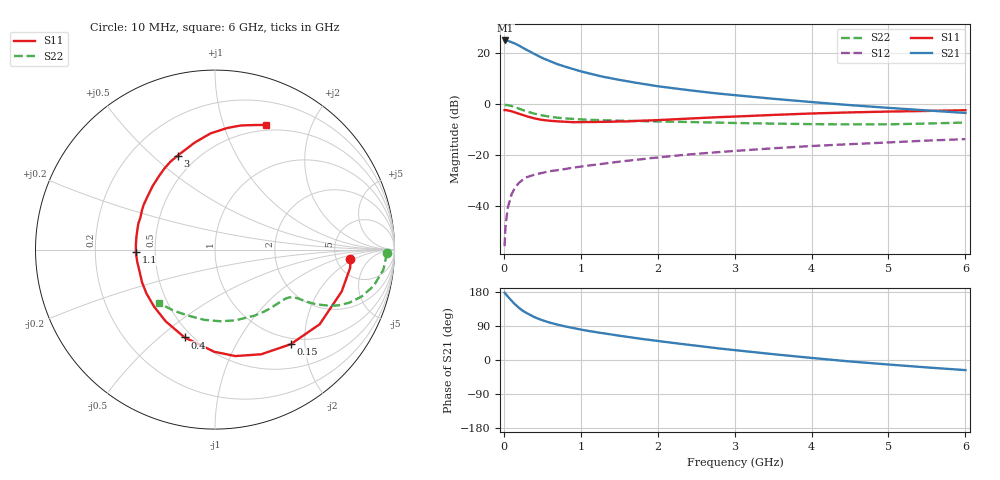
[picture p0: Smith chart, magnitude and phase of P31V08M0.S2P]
! SIEMENS Small Signal Semiconductors
! BFP181
! Si NPN RF Bipolar Junction Transistor in SOT143
! VCE = 1 V  IC = 8 mA
! Common Emitter S-Parameters:  March  1996
# GHz  S  MA  R  50
!  f  S11  S21  S12  S22
! GHz  MAG  ANG  MAG  ANG  MAG  ANG  MAG  ANG
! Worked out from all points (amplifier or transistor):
!   36 points, 10 MHz to 6 GHz, reference 50 ohm
!   highest |S21| = 24.9 dB at 20 MHz (marker M1)
!   |S21| within 3 dB of that: start of sweep to 253.4 MHz
!   unconditionally stable (mu >= 1): 794.9 MHz to end of sweep
!   at 250 MHz: K = 0.40, MSG = 25.9 dB, |S12| = -29.7 dB
!   at 1.4 GHz: K = 1.31, MAG = 13.2 dB, |S12| = -23.1 dB
!   at 6 GHz: K = 1.21, MAG = 2.4 dB, |S12| = -13.8 dB
!   S11 on the Smith chart (normalised r, x): 10 MHz: 6.80, -1.59; 150 MHz: 0.89, -1.72; 400 MHz: 0.46, -0.61; 1.1 GHz: 0.39, -0.01; 3 GHz: 0.39, +0.60; 6 GHz: 0.44, +1.40
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0.01  0.7555 -3.8  17.58 177.7  0.0016 80.5  0.9581 -1.2
0.02  0.76 -7.6  17.65 175.4  0.0037 83.9  0.9538 -2.6
0.05  0.7435 -18.3  17.33 167.9  0.0089 82.4  0.9449 -6.8
0.1  0.7163 -35.5  16.32 156.4  0.0167 72.4  0.9078 -12.8
0.15  0.675 -51.4  15.19 146.1  0.0233 64.2  0.8572 -17.8
0.2  0.6374 -66.2  13.94 137.1  0.0284 59.9  0.8045 -21.6
0.25  0.6039 -79.2  12.57 129.4  0.0326 55.1  0.7531 -24.4
0.3  0.5692 -90.4  11.47 123.5  0.0364 51.6  0.7085 -26.2
0.4  0.5181 -109.1  9.526 112.9  0.0407 47.3  0.6412 -28.4
0.5  0.4848 -124.6  7.989 104.9  0.0441 44.4  0.5929 -29.5
0.6  0.4652 -136.7  6.915 98.6  0.0476 43.7  0.559 -30.1
0.7  0.4536 -147.4  6.014 93.2  0.0499 43.3  0.535 -30.5
0.9  0.4375 -164.1  4.841 84.5  0.056 43.2  0.5068 -31.7
1.1  0.441 -178.1  4.004 76.7  0.0615 43.5  0.4879 -33.3
1.5  0.4512 161.1  2.97 64.0  0.0731 44.1  0.4683 -37.5
1.8  0.4686 148.4  2.484 55.5  0.082 43.9  0.4584 -41.8
2.2  0.4963 134.4  2.035 45.1  0.0949 42.5  0.4465 -48.1
3  0.5635 111.7  1.487 26.1  0.119 38.3  0.4211 -62.9
3.5  0.6067 100.8  1.262 15.4  0.1342 35.2  0.4104 -73.9
4.5  0.6807 84.3  0.946 -3.9  0.1616 27.7  0.3959 -98.7
5.5  0.7272 72.6  0.744 -19.6  0.19 20.6  0.4109 -123.9
6  0.751 67.7  0.664 -26.7  0.2032 16.5  0.4304 -136.1
